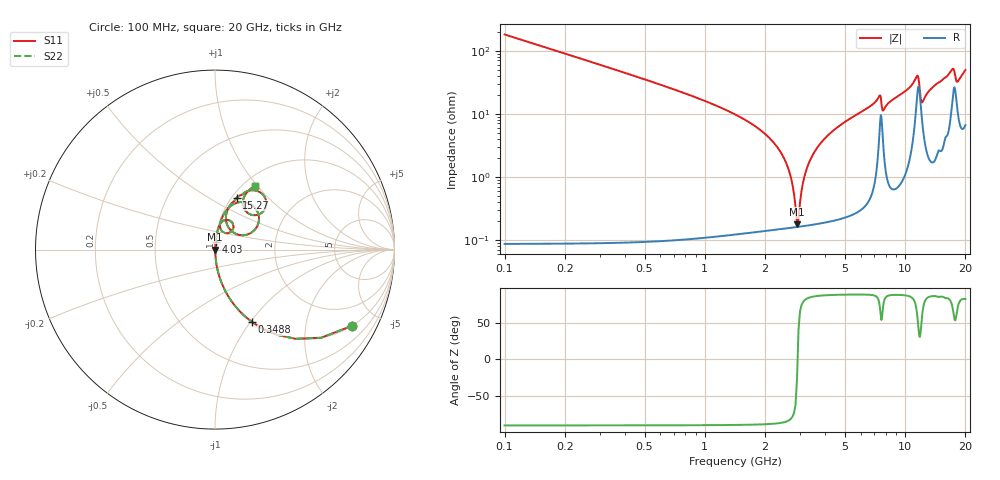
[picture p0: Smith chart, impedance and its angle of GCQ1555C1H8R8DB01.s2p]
!Murata Part Number: GCQ1555C1H8R8DB01
!These Parameters are Measured in Series Mode Connection
!Data Generated on Jan 08, 2026
!  o--ll--o
!Port1  Port2
!  o------o
!Operation Temp=25[degC], DC Bias Voltage=0[V]
!Freq. Start=100[MHz] Stop=20[GHz] 401[Steps]
# Hz S RI R 50
!Freq.(Hz) S11(Real) S11(Imag) S21(Real) S21(Imag) S12(Real) S12(Imag) S22(Real) S22(Imag)
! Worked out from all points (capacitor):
!   401 points, 100 MHz to 20 GHz, reference 50 ohm
!   read as one part in series: C = 8.8 pF near 199.5 MHz
!   lowest |Z| = 177 mohm at 2.886 GHz (marker M1)
!   series resonance near 2.904 GHz, so ESL is about 340 pH
!   S11 on the Smith chart (normalised r, x): 100 MHz: 1.00, -3.61; 348.8 MHz: 1.00, -1.02; 4.03 GHz: 1.00, +0.08; 15.27 GHz: 1.05, +0.68; 20 GHz: 1.13, +0.98
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1e8  0.7653 -0.4236  0.2347 0.4236  0.2347 0.4236  0.7653 -0.4236
3.4875e8  0.2075 -0.4047  0.7925 0.4047  0.7925 0.4047  0.2075 -0.4047
8.4625e8  0.0377 -0.188  0.9623 0.188  0.9623 0.188  0.0377 -0.188
2.33875e9  0.0022 -0.0272  0.9978 0.0272  0.9978 0.0272  0.0022 -0.0272
2.63725e9  0.00168 -0.012  0.9983 0.012  0.9983 0.012  0.00168 -0.012
2.886e9  0.00159 -0.00077  0.9984 0.00077  0.9984 0.00077  0.00159 -0.00077
2.9855e9  0.00163 0.00348  0.9984 -0.00348  0.9984 -0.00348  0.00163 0.00348
3.1845e9  0.0018 0.0116  0.9982 -0.0116  0.9982 -0.0116  0.0018 0.0116
3.43325e9  0.00217 0.0212  0.9978 -0.0212  0.9978 -0.0212  0.00217 0.0212
4.03025e9  0.00367 0.0422  0.9963 -0.0422  0.9963 -0.0422  0.00367 0.0422
6.7665e9  0.0224 0.1309  0.9776 -0.1309  0.9776 -0.1309  0.0224 0.1309
7.463e9  0.0817 0.1624  0.9183 -0.1624  0.9183 -0.1624  0.0817 0.1624
7.81125e9  0.0367 0.105  0.9633 -0.105  0.9633 -0.105  0.0367 0.105
1.005e10  0.0594 0.2132  0.9406 -0.2132  0.9406 -0.2132  0.0594 0.2132
1.149275e10  0.2292 0.2245  0.7708 -0.2245  0.7708 -0.2245  0.2292 0.2245
1.21395e10  0.0877 0.1077  0.9123 -0.1077  0.9123 -0.1077  0.0877 0.1077
1.338325e10  0.0701 0.2216  0.9299 -0.2216  0.9299 -0.2216  0.0701 0.2216
1.527375e10  0.1212 0.2899  0.8788 -0.2899  0.8788 -0.2899  0.1212 0.2899
1.67165e10  0.2007 0.3303  0.7993 -0.3303  0.7993 -0.3303  0.2007 0.3303
1.746275e10  0.2861 0.2594  0.7139 -0.2594  0.7139 -0.2594  0.2861 0.2594
1.81095e10  0.178 0.2076  0.822 -0.2076  0.822 -0.2076  0.178 0.2076
2e10  0.2252 0.3558  0.7748 -0.3558  0.7748 -0.3558  0.2252 0.3558
